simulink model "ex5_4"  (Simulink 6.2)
settings: Solver=ode3  SolverMode=SingleTasking  StartTime=0.0  StopTime=200  FixedStep=0.05  RelTol=1e-3  AbsTol=1e-6
libraries: simulink x1

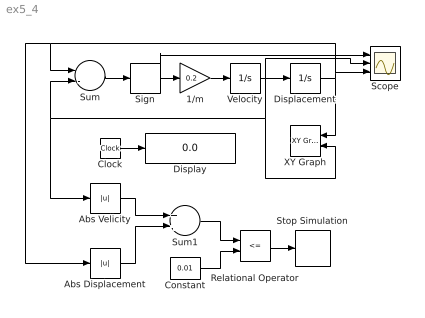
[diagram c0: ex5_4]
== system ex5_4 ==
  1/m : Gain  Gain=0.2
  Abs Displacement : Abs
  Abs Velicity : Abs
  Clock : Clock
  Constant : Constant  Value=0.01
  Displacement : Integrator  InitialCondition=1
  Display : Display
  Relational Operator : RelationalOperator  Operator=<=
  Scope : Scope  NumInputPorts=3
  Sign : Signum
  Stop Simulation : Stop
  Sum : Sum  Inputs=--
  Sum1 : Sum
  Velocity : Integrator
  XY Graph : simulink/Sinks/XY Graph  Orientation=left  xmin=-1  xmax=1  ymin=-1  ymax=1  st=-1
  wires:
  Sum/1 -> Sign/1
  Velocity/1 -> Displacement/1, Sum/2, Abs Velicity/1, XY Graph/2, Scope/2
  1/m/1 -> Velocity/1
  Displacement/1 -> XY Graph/1, Sum/1, Abs Displacement/1, Scope/3
  Relational Operator/1 -> Stop Simulation/1
  Abs Velicity/1 -> Sum1/1
  Abs Displacement/1 -> Sum1/2
  Clock/1 -> Display/1
  Sum1/1 -> Relational Operator/1
  Constant/1 -> Relational Operator/2
  Sign/1 -> 1/m/1, Scope/1
